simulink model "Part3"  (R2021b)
settings: Solver=FixedStepAuto  StartTime=0.0  StopTime=30.0  RelTol=1e-3  EnableMultiTasking=on
libraries: arduinolib x2

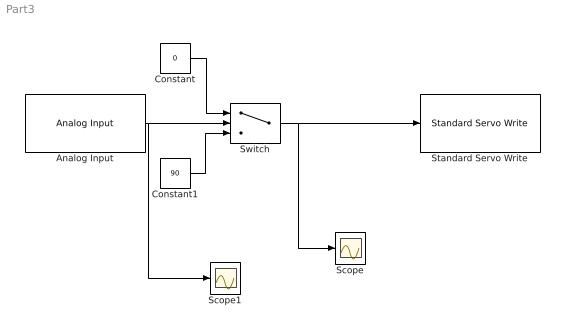
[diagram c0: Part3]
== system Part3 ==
  Analog Input : arduinolib/Analog Input  pinNumber=0  ReadResultsOnly=off  ConversionTriggerSource=Software  ExternalTriggerType=uint32( 0 )  OutputDataType=uint16  EnableConversionCompleteNotify=off  EnableOuputStatus=off  SampleTime=-1  blockPlatform=arduino
  Constant : Constant  Value=0
  Constant1 : Constant  Value=90
  Scope : Scope
  Scope1 : Scope
  Standard Servo Write : arduinolib/Standard Servo Write  pinNumber=9  ServoIndex=0  blockPlatform=ARDUINO
  Switch : Switch  Criteria=u2 > Threshold  Threshold=100
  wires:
  Constant/1 -> Switch/1
  Constant1/1 -> Switch/3
  Switch/1 -> Standard Servo Write/1, Scope/1
  Analog Input/1 -> Scope1/1, Switch/2
